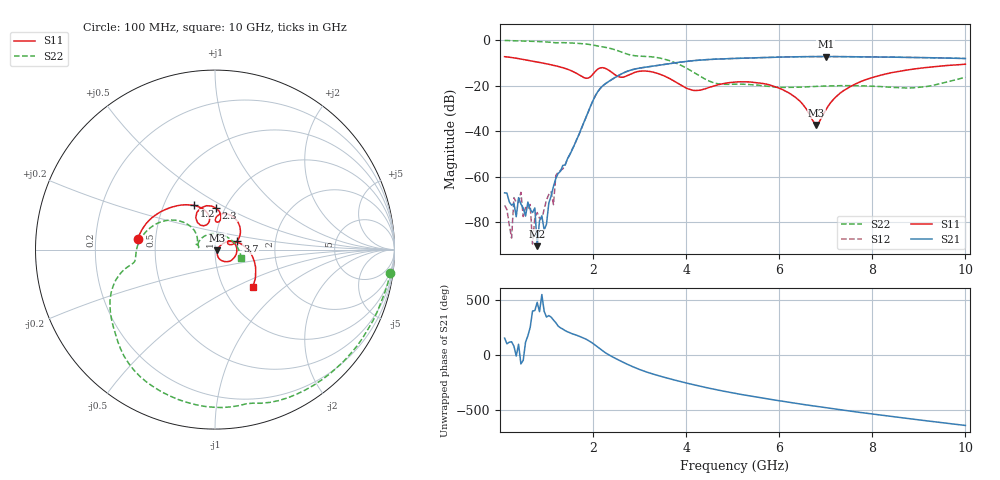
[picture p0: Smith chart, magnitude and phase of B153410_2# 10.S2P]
!  2-Port S-parameters saved by WinCal
! VAR MeasName=S-Parameters (CALIBRATED_DATA) read from VNA (N5245A)
! VAR MeasDate=2016-12-23 9:59:51
! VAR NAME=B153410_2# 10
! VAR FILENAME=B153410_2# 10.S2P
! VAR DATE=2016-12-23 9:59:51
! VAR PHYS_PORTS=1,2
# Hz S DB R 50
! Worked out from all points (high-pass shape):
!   199 points, 100 MHz to 10 GHz, reference 50 ohm
!   highest |S21| = -7.19 dB at 7 GHz (marker M1); lowest = -90.5 dB at 800 MHz (marker M2)
!   |S21| within 3 dB of the highest: 3.686 GHz to end of sweep
!   lowest |S11| = -37.2 dB at 6.8 GHz (marker M3), VSWR 1.03, Z = 51.3 - j0.361 ohm
!   |S11| at or under -10 dB: 903.8 MHz to end of sweep
!   |S22| runs from -21.0 to -0.1 dB; largest |S21 - S12| = 0.0036
!   S11 on the Smith chart (normalised r, x): 100 MHz: 0.40, +0.05; 1.2 GHz: 0.71, +0.38; 2.3 GHz: 0.91, +0.44; 3.7 GHz: 1.28, +0.13; 10 GHz: 1.37, -0.63
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1e8  -7.25 172.5  -67.06 154.0  -72.52 32.1  -0.13 -7.5
2.5e8  -7.61 162.2  -72.50 120.5  -86.93 -24.3  -0.26 -17.6
3e8  -7.75 159.0  -71.70 80.7  -69.16 -85.0  -0.28 -21.0
3.5e8  -7.93 156.0  -77.52 -9.8  -71.22 137.1  -0.31 -24.3
4e8  -8.10 153.1  -69.18 97.9  -71.24 -11.6  -0.35 -27.6
4.5e8  -8.29 150.3  -71.95 -81.8  -66.82 -5.8  -0.37 -30.9
5e8  -8.48 147.7  -73.74 -48.7  -77.46 -138.0  -0.39 -34.2
8e8  -9.61 133.4  -90.47 121.0  -75.69 -63.4  -0.59 -53.9
1e9  -10.38 124.5  -80.78 -13.2  -70.14 38.8  -0.79 -67.1
1.15e9  -11.04 117.9  -64.19 -40.9  -72.26 -26.7  -1.10 -76.1
1.2e9  -11.27 115.6  -60.79 -64.8  -59.48 -60.5  -1.14 -78.5
1.75e9  -15.83 101.2  -38.69 162.3  -38.94 162.6  -1.52 -113.6
2.3e9  -12.74 88.3  -18.64 11.0  -18.62 11.2  -3.30 -148.3
3.4e9  -14.68 40.6  -11.08 171.4  -11.08 171.5  -7.74 169.3
3.7e9  -17.50 21.3  -10.15 136.6  -10.14 136.7  -9.39 153.0
5.05e9  -18.40 7.0  -8.02 9.4  -8.04 9.6  -19.32 163.4
6.05e9  -21.51 -52.3  -7.41 -61.7  -7.41 -61.6  -20.71 169.0
6.7e9  -34.58 -50.7  -7.20 -103.8  -7.22 -103.7  -20.38 171.7
6.8e9  -37.23 -14.8  -7.19 -110.0  -7.21 -109.9  -20.26 171.1
7e9  -30.64 34.2  -7.19 -122.2  -7.21 -122.1  -20.16 168.6
8.35e9  -14.55 -1.1  -7.45 161.1  -7.44 161.5  -20.62 118.4
1e10  -10.56 -44.6  -8.06 75.8  -8.05 76.3  -16.28 -16.8
